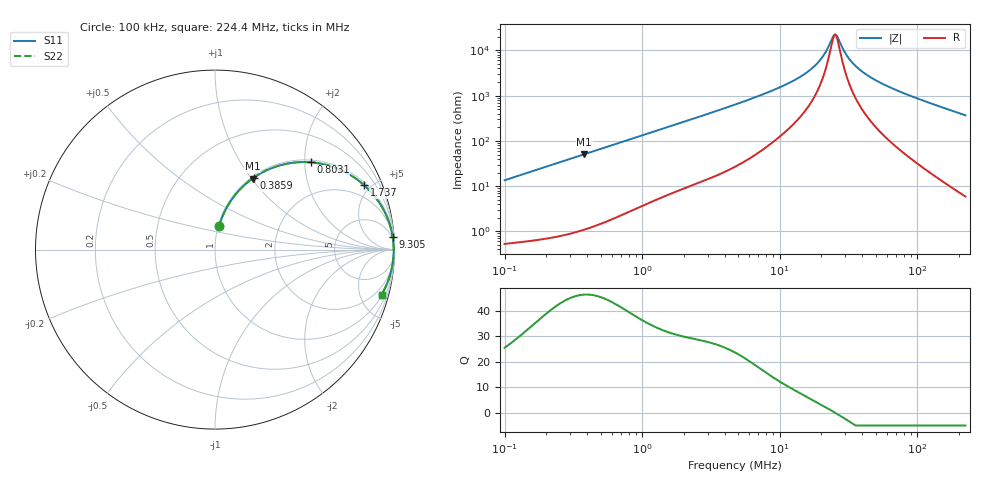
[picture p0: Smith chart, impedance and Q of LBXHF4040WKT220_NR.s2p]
! LBXHF4040WKT220_NR  S-PARAMETER MODEL  ( General Type )
! Model Generated by TAIYO YUDEN Corporation (http://www.ty-top.com)
! Version 1.0
! TAIYO YUDEN Control No. 210719NI43SB-FBB
! Copyright(c) 2021 TAIYO YUDEN CO.,LTD. All Rights Reserved.
! Product Description (link to TY-COMPAS)
! https://ds.yuden.co.jp/TYCOMPAS/or/detail?pn=LBXHF4040WKT220MNR&u=M
! Products Name : Inductors
! Characteristics :
!  Inductance : 22 uH , SRF(min) : 17 MHz , DC Resistance(max) : 0.36 Ohm
!  Rated Current : Saturation :1000 mA , Temp Rise : 710 mA
!  Case Size : 4.0 x 4.0 / 0.157 x 0.157 [mm/inch] , Thickness : 2 / 0.079 [mm/inch]
!  (Conditions: Temperature = 25 degC , DC Bias Current/Voltage = 0A / 0V)
! External Node Assignments :
!  1  o---GGG---o  2
! GND o---------o GND
! Frequency Range : 0.1MHz  -  224.402193MHz  [ 402 STEP ]
# MHz S RI R 50
! Freq[MHz].  S11 Real  S11 Imag  S21 Real  S21 Imag  S12 Real  S12 Imag  S22 Real  S22 Imag
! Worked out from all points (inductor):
!   401 points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, 100 kHz to 224.4 MHz, reference 50 ohm
!   read as one part in series: L = 21.4 uH near 103.9 kHz
!   highest Q = 46.4 at 378.5 kHz (marker M1), where L = 21.3 uH
!   self-resonance near 24.89 MHz
!   S11 on the Smith chart (normalised r, x): 100 kHz: 1.01, +0.27; 385.9 kHz: 1.02, +1.03; 803.1 kHz: 1.05, +2.14; 1.737 MHz: 1.15, +4.58; 9.305 MHz: 3, +28; 224.4 MHz: 1.12, -7.37
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0.1  0.0229 0.1311  0.9771 -0.1311  0.9771 -0.1311  0.0229 0.1311
0.208136  0.0778 0.2555  0.9222 -0.2555  0.9222 -0.2555  0.0778 0.2555
0.364164  0.1969 0.387  0.8031 -0.387  0.8031 -0.387  0.1969 0.387
0.378488  0.209 0.3959  0.791 -0.3959  0.791 -0.3959  0.209 0.3959
0.38586  0.2152 0.4004  0.7848 -0.4004  0.7848 -0.4004  0.2152 0.4004
0.803114  0.5322 0.4865  0.4678 -0.4865  0.4678 -0.4865  0.5322 0.4865
1.326154  0.748 0.4193  0.252 -0.4193  0.252 -0.4193  0.748 0.4193
1.737321  0.8318 0.3582  0.1682 -0.3582  0.1682 -0.3582  0.8318 0.3582
4.737111  0.9697 0.1516  0.0303 -0.1516  0.0303 -0.1516  0.9697 0.1516
9.305258  0.9896 0.0709  0.0104 -0.0709  0.0104 -0.0709  0.9896 0.0709
13.42463  0.9933 0.0412  0.00671 -0.0412  0.00671 -0.0412  0.9933 0.0412
17.25085  0.9947 0.024  0.00531 -0.024  0.00531 -0.024  0.9947 0.024
20.52148  0.9953 0.013  0.00474 -0.013  0.00474 -0.013  0.9953 0.013
24.41219  0.9956 0.00226  0.00445 -0.00226  0.00445 -0.00226  0.9956 0.00226
25.37242  0.9956 -0.000104  0.00442 0.000104  0.00442 0.000104  0.9956 -0.000104
26.37042  0.9956 -0.00247  0.0044 0.00247  0.0044 0.00247  0.9956 -0.00247
31.37005  0.9955 -0.0132  0.00449 0.0132  0.00449 0.0132  0.9955 -0.0132
35.90527  0.9953 -0.0219  0.00475 0.0219  0.00475 0.0219  0.9953 -0.0219
45.25733  0.9944 -0.0377  0.00564 0.0377  0.00564 0.0377  0.9944 -0.0377
62.8214  0.9917 -0.0636  0.00826 0.0636  0.00826 0.0636  0.9917 -0.0636
109.915  0.98 -0.1244  0.02 0.1244  0.02 0.1244  0.98 -0.1244
224.4022  0.9279 -0.2508  0.0721 0.2508  0.0721 0.2508  0.9279 -0.2508
